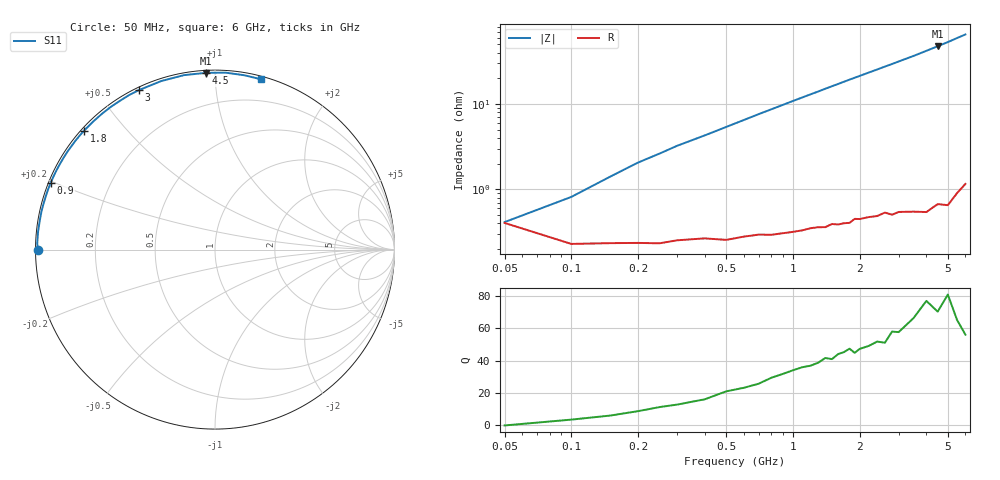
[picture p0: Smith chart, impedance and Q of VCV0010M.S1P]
! Infineon Technologies  Discrete & RF Semiconductors
! BBY 56-03
! Si Tuning Diode in SOD323
! VR =
! S-Parameters:  June  1999
# GHz  S  MA  R  50
!  f  S11
! GHz  MAG  ANG
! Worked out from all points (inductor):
!   34 points, 50 MHz to 6 GHz, reference 50 ohm
!   read as one part to ground: L = 1.48 nH near 100 MHz
!   highest Q = 77 at 4.5 GHz (marker M1), where L = 1.68 nH
!   S11 on the Smith chart (normalised r, x): 50 MHz: 0.01, -0.00; 900 MHz: 0.01, +0.20; 1.8 GHz: 0.01, +0.39; 3 GHz: 0.01, +0.63; 4.5 GHz: 0.01, +0.95; 6 GHz: 0.02, +1.30
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0.05  0.9839 -179.8
0.1  0.9908 178.2
0.15  0.9906 176.8
0.2  0.9906 175.3
0.3  0.9899 172.6
0.5  0.9899 167.7
0.7  0.9885 162.7
0.8  0.9886 160.3
0.9  0.9882 157.9
1  0.9879 155.5
1.2  0.9869 150.9
1.3  0.9867 148.7
1.4  0.9868 146.4
1.6  0.9862 142.1
1.7  0.9859 139.9
1.8  0.9859 137.8
2  0.9849 133.8
2.2  0.9845 129.9
2.4  0.9846 126.2
2.6  0.9836 122.5
2.8  0.985 119.1
3  0.9845 115.6
3.5  0.9858 107.7
4  0.9873 100.0
4.5  0.9859 93.0
5  0.9878 86.6
5.5  0.985 80.4
6  0.9829 75.0
